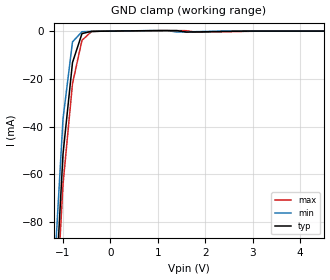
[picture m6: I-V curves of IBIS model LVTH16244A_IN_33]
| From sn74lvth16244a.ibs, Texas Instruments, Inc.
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|   Model LVTH16244A Input_IN_33
[Model]   LVTH16244A_IN_33
Model_type  Input
Polarity   Inverting
Vinl = 0.8V
Vinh = 2.0V
| variable   typ   min   max
C_comp   4pf   NA   NA
[Temperature Range]   40   -25   100
| Ambient temperature   25   -40   85
[Voltage range]   3.3   3.0   3.6
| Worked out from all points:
|   GND clamp passes 1 mA (typ) near -0.59 V on its own axis
[GND Clamp]
|   Voltage   I(typ)   I(min)   I(max)
-5V       -2.136A    -2.461A    -1.908A
-1.2V     -125.6mA   -106.7mA   -137.1mA
-1V       -51.48mA   -36.78mA   -64.25mA
-800mV    -13.18mA   -4.517mA   -21.98mA
-600mV    -1.05mA    -258uA     -3.859mA
-400mV    -102.8uA   -113.1uA   -220.8uA
-200mV    -48.38uA   -55.42uA   -43.75uA
1.2V      220.1uA    229.6uA    207.8uA
1.4V      197.9uA    -369.8uA   215.3uA
1.6V      -405.3uA   -309uA     175uA
1.8V      -353.5uA   -236.3uA   -437uA
5V        -26.46pA   3.76uA     645.8pA
